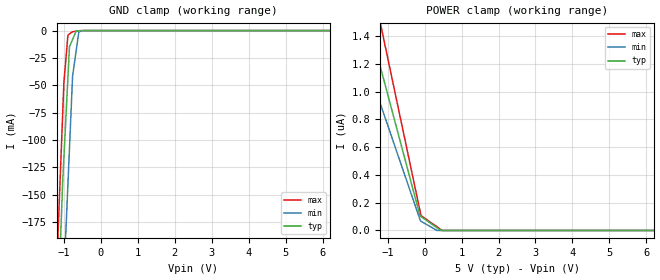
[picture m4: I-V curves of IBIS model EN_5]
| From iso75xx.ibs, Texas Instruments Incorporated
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|   EN_5 Model
[Model]   EN_5
Model_type   Input
Vinl = .8
Vinh = 2
|   typ   min   max
|   (typ PVT)   (Fast PVT)   (Slow PVT)
C_comp   0.4382p   0.3816p   0.5008p
[Voltage Range]   5   4.5   5.5
[Temperature Range]   27   125   -40
[Power Clamp Reference]   5   4.5   5.5
[GND Clamp Reference]   -0   -0   -0
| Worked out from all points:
|   GND clamp passes 1 mA (typ) near -0.68 V on its own axis
[GND Clamp]
|   Voltage   I(typ)   I(min)   I(max)
-5V       -4.018A    -4.118A    -3.957A
-1.301V   -380.5mA   -493mA     -308.8mA
-1.065V   -167.4mA   -276.3mA   -103.9mA
-1.033V   -138mA     -250.9mA   -75.61mA
-1.001V   -116.3mA   -225.7mA   -47.61mA
-891.9mV  -43mA      -140.6mA   -4.255mA
-850.3mV  -14.96mA   -108.1mA   -3.132mA
-783.1mV  -9.544mA   -55.51mA   -1.318mA
-765.4mV  -8.116mA   -41.64mA   -1.173mA
-596.6mV  -178.1uA   -1.14mA    -169.1uA
-475.6mV  -60.57uA   -52.81uA   -19.55uA
10V       0A         0A         0A
[POWER Clamp]
|   Voltage   I(typ)   I(min)   I(max)
-5V       4.99uA     3.885uA    6.297uA
-4.902V   4.875uA    3.791uA    6.157uA
-1.033V   1.013uA    783.7nA    1.284uA
-122.8mV  104.7nA    76.34nA    138nA
-98.1mV   100.1nA    66.19nA    106.9nA
335.5mV   19.35nA    0A         26.11nA
439.4mV   0A         0A         6.747nA
475.6mV   0A         0A         0A
10V       0A         0A         0A
